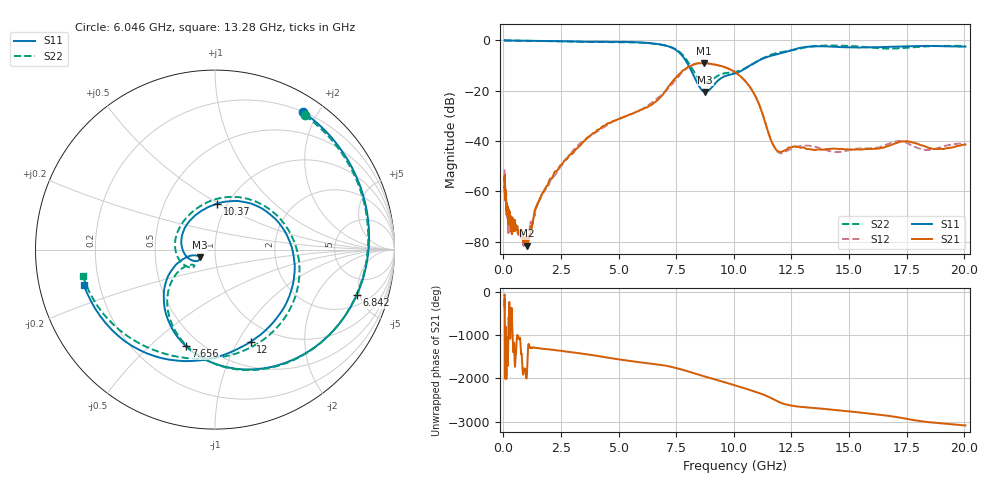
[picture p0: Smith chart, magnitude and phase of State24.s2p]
# Hz S DB R 50
!freq MagS11 AngS11 MagS21 AngS21 MagS12 AngS12 MagS22 AngS22
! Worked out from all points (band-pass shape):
!   1601 points, 50 MHz to 20.05 GHz, reference 50 ohm
!   highest |S21| = -8.95 dB at 8.696 GHz (marker M1); lowest = -81.6 dB at 1.024 GHz (marker M2)
!   |S21| within 3 dB of the highest: 7.785 GHz to 9.937 GHz (2.152 GHz wide, 24.3 % of centre)
!   lowest |S11| = -20.4 dB at 8.761 GHz (marker M3), VSWR 1.21, Z = 42 - j3.62 ohm
!   |S11| at or under -10 dB: 8.037 GHz to 10.69 GHz (2.654 GHz wide, 28.3 % of centre)
!   |S22| runs from -16.8 to 0.0 dB; largest |S21 - S12| = 0.024
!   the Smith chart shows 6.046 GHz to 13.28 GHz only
!   S11 on the Smith chart (normalised r, x): 6.046 GHz: 0.20, +1.81; 6.842 GHz: 2.87, -4.67; 7.656 GHz: 0.42, -0.66; 10.37 GHz: 0.90, +0.49; 12 GHz: 0.77, -1.13; 13.28 GHz: 0.14, -0.13
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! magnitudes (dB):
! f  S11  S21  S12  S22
! 50 MHz  0.0  -55.5  -51.3  0.0
! 62.13 MHz  0.0  -55.2  -61.7  0.0
! 101.9 MHz  0.0  -60.3  -59.8  0.0
! 135.9 MHz  0.0  -65.6  -67.6  0.0
! 187.6 MHz  0.0  -69.8  -69.1  0.0
! 209.2 MHz  0.0  -73.1  -76.2  0.0
! 244.8 MHz  0.0  -67.9  -69.9  0.0
! 369.6 MHz  0.0  -76.4  -73.6  0.0
! 495.1 MHz  0.0  -71.6  -73.6  -0.1
! 1.005 GHz  -0.1  -79.4  -79.3  -0.1
! 1.024 GHz  -0.1  -81.6  -80.7  -0.1
! 2.722 GHz  -0.3  -47.3  -47.2  -0.4
! 6.046 GHz  -0.8  -27.3  -27.2  -0.9
! 6.842 GHz  -1.6  -22.3  -21.8  -1.7
! 7.402 GHz  -3.3  -15.6  -16.4  -3.1
! 7.656 GHz  -5.0  -13.2  -13.8  -4.6
! 8.696 GHz  -20.3  -8.9  -8.9  -16.7
! 8.761 GHz  -20.4  -9.0  -8.9  -16.8
! 10.37 GHz  -11.8  -15.0  -15.0  -11.6
! 12 GHz  -5.2  -44.3  -44.8  -4.7
! 13.28 GHz  -2.4  -43.2  -41.9  -2.5
! 20.05 GHz  -2.4  -41.4  -41.0  -2.1
